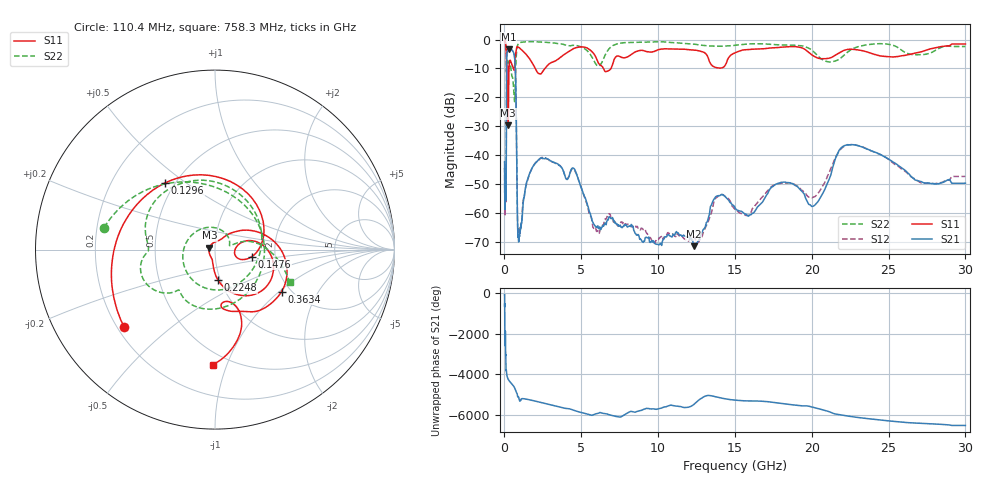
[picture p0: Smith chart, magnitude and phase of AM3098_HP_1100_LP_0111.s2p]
! Date/Time: Thu, Feb 28, 2019 8:44 AM
! Network Analyzer: Agilent Technologies E8364B Rev: A.07.50.67
! Sweep from 0.010 to 30.000 GHz, 1601 Points, Sweep Type: LOG
! Power Supply: 5.023 V, 0.002 A
# Hz S DB R 50
!freq MagS11 AngS11 MagS21 AngS21 MagS12 AngS12 MagS22 AngS22
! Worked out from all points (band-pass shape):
!   1601 points, 10 MHz to 30 GHz, reference 50 ohm
!   highest |S21| = -3.43 dB at 265.1 MHz (marker M1); lowest = -71.4 dB at 12.31 GHz (marker M2)
!   |S21| within 3 dB of the highest: 148.6 MHz to 664.8 MHz (516.3 MHz wide, 127 % of centre)
!   lowest |S11| = -29.6 dB at 246 MHz (marker M3), VSWR 1.07, Z = 47 + j1.01 ohm
!   |S11| at or under -10 dB: 205.3 MHz to 297.6 MHz (92.29 MHz wide, 36.7 % of centre); 2.008 GHz to 2.642 GHz (633.8 MHz wide, 27.3 % of centre); 6.447 GHz to 6.931 GHz (484 MHz wide, 7.24 % of centre)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
!   |S22| runs from -21.5 to -0.5 dB; largest |S21 - S12| = 0.012
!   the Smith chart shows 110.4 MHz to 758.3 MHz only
!   S11 on the Smith chart (normalised r, x): 110.4 MHz: 0.23, -0.35; 129.6 MHz: 0.44, +0.42; 147.6 MHz: 1.51, -0.12; 224.8 MHz: 0.98, -0.35; 363.4 MHz: 1.79, -1.04; 758.3 MHz: 0.41, -0.89
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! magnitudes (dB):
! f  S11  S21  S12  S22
! 10 MHz  -0.4  -42.2  -44.8  -0.5
! 38.04 MHz  -0.4  -56.6  -57.5  -0.8
! 110.4 MHz  -3.5  -50.8  -50.1  -4.0
! 129.6 MHz  -6.7  -21.4  -21.4  -10.9
! 144.7 MHz  -11.8  -7.6  -7.6  -9.6
! 147.6 MHz  -13.6  -6.7  -6.6  -9.9
! 224.8 MHz  -15.3  -3.6  -3.6  -8.2
! 246 MHz  -29.6  -3.5  -3.4  -8.6
! 265.1 MHz  -17.1  -3.4  -3.4  -8.5
! 363.4 MHz  -7.2  -3.7  -3.7  -7.8
! 550.5 MHz  -9.6  -4.1  -4.1  -13.9
! 662.4 MHz  -9.6  -6.3  -6.3  -21.5
! 758.3 MHz  -3.8  -22.4  -22.4  -6.9
! 846.5 MHz  -2.5  -61.8  -61.2  -2.1
! 907.9 MHz  -2.6  -68.8  -66.5  -1.5
! 2.084 GHz  -10.8  -42.3  -42.2  -0.8
! 7.926 GHz  -6.2  -64.1  -64.0  -1.1
! 12.31 GHz  -3.6  -71.4  -68.3  -1.6
! 13.95 GHz  -9.9  -54.0  -53.9  -2.3
! 20.31 GHz  -6.2  -56.6  -53.8  -5.2
! 22.56 GHz  -3.4  -36.3  -36.3  -3.5
! 30 GHz  -1.6  -49.7  -47.3  -2.4
